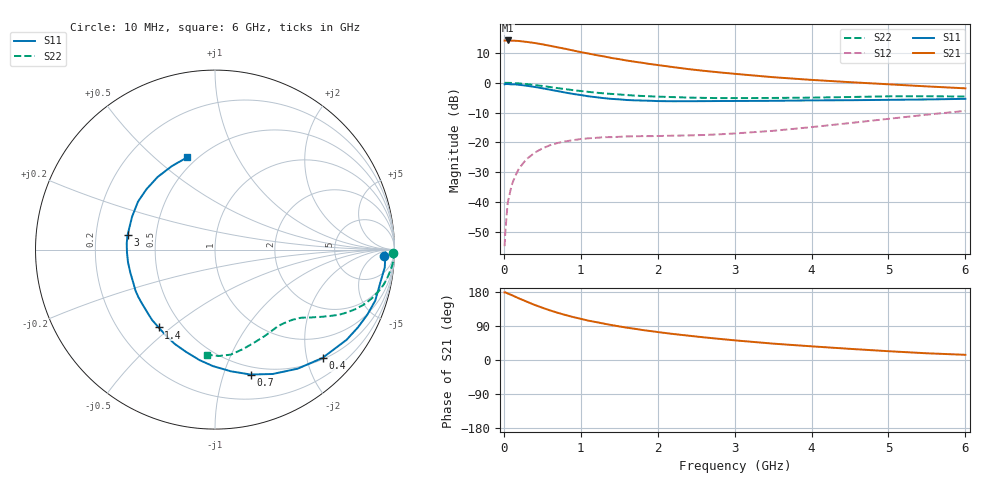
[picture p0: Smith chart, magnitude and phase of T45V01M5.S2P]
! Infineon Technologies  Discrete & RF Semiconductors
! BFR182T
! Si NPN RF Bipolar Junction Transistor in SC75
! VCE = 5 V  IC = 1.5 mA
! Common Emitter S-Parameters:  October  1999
# GHz  S  MA  R  50
!  f  S11  S21  S12  S22
! GHz  MAG  ANG  MAG  ANG  MAG  ANG  MAG  ANG
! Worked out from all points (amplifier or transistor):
!   36 points, 10 MHz to 6 GHz, reference 50 ohm
!   highest |S21| = 14.2 dB at 50 MHz (marker M1)
!   |S21| within 3 dB of that: start of sweep to 834.2 MHz
!   unconditionally stable (mu >= 1): 2.209 GHz to 4.453 GHz
!   at 250 MHz: K = 0.11, MSG = 20.5 dB, |S12| = -27.1 dB
!   at 1.4 GHz: K = 0.68, MSG = 13.3 dB, |S12| = -18.3 dB
!   at 6 GHz: K = 0.83, MSG = 3.8 dB, |S12| = -9.4 dB
!   S11 on the Smith chart (normalised r, x): 10 MHz: 23, -14; 400 MHz: 0.53, -2.30; 700 MHz: 0.42, -1.23; 1.4 GHz: 0.37, -0.45; 3 GHz: 0.34, +0.07; 6 GHz: 0.45, +0.64
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0.01  0.9396 -2.2  5.1 178.5  0.0018 79.1  0.9901 -1.2
0.02  0.9507 -0.9  5.102 178.6  0.0032 93.6  0.9961 -1.0
0.05  0.9509 -6.0  5.129 175.5  0.0096 88.1  0.9957 -2.4
0.1  0.9392 -11.3  5.093 171.5  0.0188 83.6  0.9924 -4.7
0.2  0.9227 -23.2  5.016 162.3  0.0367 78.2  0.9735 -9.2
0.3  0.889 -34.4  4.843 153.7  0.0527 71.3  0.9488 -13.4
0.4  0.8504 -45.2  4.649 145.4  0.0667 65.1  0.9161 -17.2
0.5  0.8078 -55.2  4.417 138.0  0.0788 59.9  0.8827 -20.4
0.6  0.764 -65.1  4.174 130.9  0.0891 55.8  0.8466 -23.2
0.7  0.7237 -74.1  3.932 124.6  0.0975 51.8  0.8125 -25.6
0.9  0.6489 -91.1  3.48 113.4  0.1086 45.9  0.7503 -29.4
1.1  0.5916 -106.0  3.094 103.8  0.1167 41.5  0.7025 -32.2
1.4  0.5355 -125.9  2.608 92.2  0.1221 37.7  0.6488 -35.7
1.6  0.5126 -138.1  2.36 85.3  0.1254 36.7  0.621 -37.6
1.8  0.5021 -148.5  2.162 79.2  0.1269 36.5  0.5991 -39.8
2.2  0.4889 -164.9  1.83 68.7  0.1291 38.3  0.5739 -43.9
2.6  0.4908 -178.3  1.585 59.8  0.1326 41.9  0.5566 -48.7
3  0.4939 170.7  1.412 51.9  0.1406 46.2  0.552 -53.3
3.5  0.4969 158.5  1.239 43.2  0.1558 51.9  0.5554 -60.1
4.5  0.509 138.6  1.022 29.4  0.2104 58.6  0.5757 -74.2
5.5  0.5238 117.2  0.868 17.7  0.291 58.4  0.5934 -88.2
6  0.5365 106.9  0.805 13.7  0.3369 55.7  0.5865 -94.6
